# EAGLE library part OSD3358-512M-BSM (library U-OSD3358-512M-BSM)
Octavo Systems LLC OSD335x Family SiP: 21mm x 21mm, 1.27mm pitch 256 pin BGA contains AM3358, 512MB DDR3, TPS65217, TL5209, 4KB EEPROM and passives. Commerical Temperature (case): 0C to 85C.
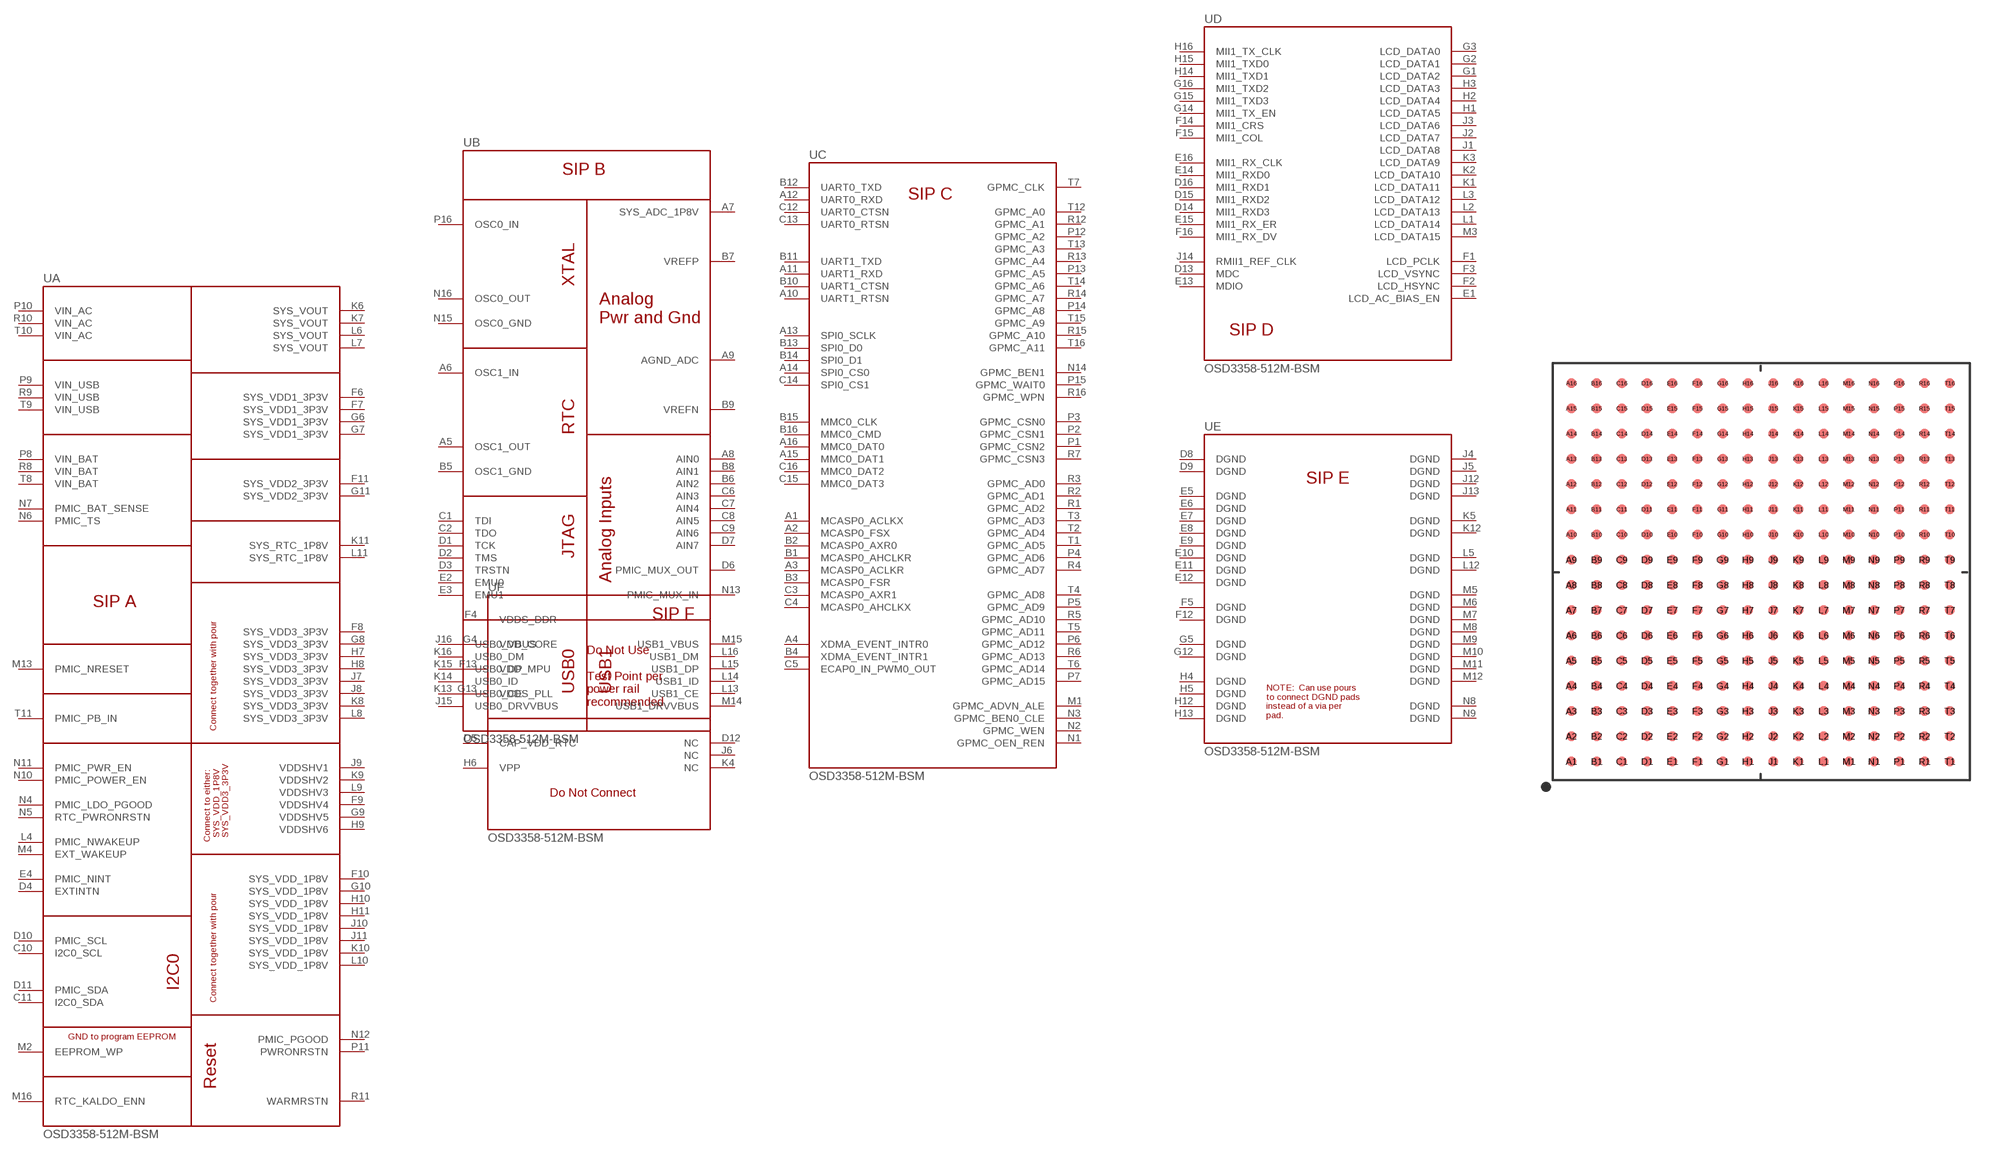
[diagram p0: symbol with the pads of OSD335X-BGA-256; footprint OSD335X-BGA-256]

Designator prefix U; gates A=OSD335X-SM-LOGICAL-A B=OSD335X-SM-LOGICAL-B C=OSD335X-SM-LOGICAL-C D=OSD335X-SM-LOGICAL-D E=OSD335X-SM-LOGICAL-E F=OSD335X-SM-LOGICAL-F

## OSD3358-512M-BSM (DESCRIPTION: 21mm 256 Ball Bga; DIGI-KEY_PART_NUMBER: 1676-1002-ND; DIGI-KEY_PURCHASE_URL: https://www.digikey.com/product-detail/en/octavo-systems-llc/OSD3358-512M-BSM/1676-1002-ND/7644258?utm_source=snapeda&utm_medium=aggregator&utm_campaign=symbol; MF: Octavo Systems; MP: OSD3358-512M-BSM; PACKAGE: BGA-400 Octavo Systems)  [OSD335X-BGA-256]
A1  C:MCASP0_ACLKX
A2  C:MCASP0_FSX
A3  C:MCASP0_ACLKR
A4  C:XDMA_EVENT_INTR0
A5  B:OSC1_OUT
A6  B:OSC1_IN
A7  B:SYS_ADC_1P8V
A8  B:AIN0
A9  B:AGND_ADC
A10  C:UART1_RTSN
A11  C:UART1_RXD
A12  C:UART0_RXD
A13  C:SPI0_SCLK
A14  C:SPI0_CS0
A15  C:MMC0_DAT1
A16  C:MMC0_DAT0
B1  C:MCASP0_AHCLKR
B2  C:MCASP0_AXR0
B3  C:MCASP0_FSR
B4  C:XDMA_EVENT_INTR1
B5  B:OSC1_GND
B6  B:AIN2
B7  B:VREFP
B8  B:AIN1
B9  B:VREFN
B10  C:UART1_CTSN
B11  C:UART1_TXD
B12  C:UART0_TXD
B13  C:SPI0_D0
B14  C:SPI0_D1
B15  C:MMC0_CLK
B16  C:MMC0_CMD
C1  B:TDI
C2  B:TDO
C3  C:MCASP0_AXR1
C4  C:MCASP0_AHCLKX
C5  C:ECAP0_IN_PWM0_OUT
C6  B:AIN3
C7  B:AIN4
C8  B:AIN5
C9  B:AIN6
C10  A:I2C0_SCL
C11  A:I2C0_SDA
C12  C:UART0_CTSN
C13  C:UART0_RTSN
C14  C:SPI0_CS1
C15  C:MMC0_DAT3
C16  C:MMC0_DAT2
D1  B:TCK
D2  B:TMS
D3  B:TRSTN
D4  A:EXTINTN
D5  F:CAP_VDD_RTC
D6  B:PMIC_MUX_OUT
D7  B:AIN7
D8  E:DGND
D9  E:DGND
D10  A:PMIC_SCL
D11  A:PMIC_SDA
D12  F:NC
D13  D:MDC
D14  D:MII1_RXD3
D15  D:MII1_RXD2
D16  D:MII1_RXD1
E1  D:LCD_AC_BIAS_EN
E2  B:EMU0
E3  B:EMU1
E4  A:PMIC_NINT  out
E5  E:DGND
E6  E:DGND
E7  E:DGND
E8  E:DGND
E9  E:DGND
E10  E:DGND
E11  E:DGND
E12  E:DGND
E13  D:MDIO
E14  D:MII1_RXD0
E15  D:MII1_RX_ER
E16  D:MII1_RX_CLK
F1  D:LCD_PCLK
F2  D:LCD_HSYNC
F3  D:LCD_VSYNC
F4  F:VDDS_DDR
F5  E:DGND
F6  A:SYS_VDD1_3P3V  pwr
F7  A:SYS_VDD1_3P3V  pwr
F8  A:SYS_VDD3_3P3V  pwr
F9  A:VDDSHV4  pwr
F10  A:SYS_VDD_1P8V  pwr
F11  A:SYS_VDD2_3P3V  pwr
F12  E:DGND
F13  F:VDD_MPU
F14  D:MII1_CRS
F15  D:MII1_COL
F16  D:MII1_RX_DV
G1  D:LCD_DATA2
G2  D:LCD_DATA1
G3  D:LCD_DATA0
G4  F:VDD_CORE
G5  E:DGND
G6  A:SYS_VDD1_3P3V  pwr
G7  A:SYS_VDD1_3P3V  pwr
G8  A:SYS_VDD3_3P3V  pwr
G9  A:VDDSHV5  pwr
G10  A:SYS_VDD_1P8V  pwr
G11  A:SYS_VDD2_3P3V  pwr
G12  E:DGND
G13  F:VDDS_PLL
G14  D:MII1_TX_EN
G15  D:MII1_TXD3
G16  D:MII1_TXD2
H1  D:LCD_DATA5
H2  D:LCD_DATA4
H3  D:LCD_DATA3
H4  E:DGND
H5  E:DGND
H6  F:VPP
H7  A:SYS_VDD3_3P3V  pwr
H8  A:SYS_VDD3_3P3V  pwr
H9  A:VDDSHV6  pwr
H10  A:SYS_VDD_1P8V  pwr
H11  A:SYS_VDD_1P8V  pwr
H12  E:DGND
H13  E:DGND
H14  D:MII1_TXD1
H15  D:MII1_TXD0
H16  D:MII1_TX_CLK
J1  D:LCD_DATA8
J2  D:LCD_DATA7
J3  D:LCD_DATA6
J4  E:DGND
J5  E:DGND
J6  F:NC
J7  A:SYS_VDD3_3P3V  pwr
J8  A:SYS_VDD3_3P3V  pwr
J9  A:VDDSHV1  pwr
J10  A:SYS_VDD_1P8V  pwr
J11  A:SYS_VDD_1P8V  pwr
J12  E:DGND
J13  E:DGND
J14  D:RMII1_REF_CLK
J15  B:USB0_DRVVBUS
J16  B:USB0_VBUS
K1  D:LCD_DATA11
K2  D:LCD_DATA10
K3  D:LCD_DATA9
K4  F:NC
K5  E:DGND
K6  A:SYS_VOUT  pwr
K7  A:SYS_VOUT  pwr
K8  A:SYS_VDD3_3P3V  pwr
K9  A:VDDSHV2  pwr
K10  A:SYS_VDD_1P8V  pwr
K11  A:SYS_RTC_1P8V  pwr
K12  E:DGND
K13  B:USB0_CE
K14  B:USB0_ID
K15  B:USB0_DP
K16  B:USB0_DM
L1  D:LCD_DATA14
L2  D:LCD_DATA13
L3  D:LCD_DATA12
L4  A:PMIC_NWAKEUP  out
L5  E:DGND
L6  A:SYS_VOUT  pwr
L7  A:SYS_VOUT  pwr
L8  A:SYS_VDD3_3P3V  pwr
L9  A:VDDSHV3  pwr
L10  A:SYS_VDD_1P8V  pwr
L11  A:SYS_RTC_1P8V  pwr
L12  E:DGND
L13  B:USB1_CE
L14  B:USB1_ID
L15  B:USB1_DP
L16  B:USB1_DM
M1  C:GPMC_ADVN_ALE
M2  A:EEPROM_WP
M3  D:LCD_DATA15
M4  A:EXT_WAKEUP
M5  E:DGND
M6  E:DGND
M7  E:DGND
M8  E:DGND
M9  E:DGND
M10  E:DGND
M11  E:DGND
M12  E:DGND
M13  A:PMIC_NRESET
M14  B:USB1_DRVVBUS
M15  B:USB1_VBUS
M16  A:RTC_KALDO_ENN
N1  C:GPMC_OEN_REN
N2  C:GPMC_WEN
N3  C:GPMC_BEN0_CLE
N4  A:PMIC_LDO_PGOOD  out
N5  A:RTC_PWRONRSTN
N6  A:PMIC_TS
N7  A:PMIC_BAT_SENSE
N8  E:DGND
N9  E:DGND
N10  A:PMIC_POWER_EN  out
N11  A:PMIC_PWR_EN  in
N12  A:PMIC_PGOOD  out
N13  B:PMIC_MUX_IN
N14  C:GPMC_BEN1
N15  B:OSC0_GND
N16  B:OSC0_OUT
P1  C:GPMC_CSN2
P2  C:GPMC_CSN1
P3  C:GPMC_CSN0
P4  C:GPMC_AD6
P5  C:GPMC_AD9
P6  C:GPMC_AD12
P7  C:GPMC_AD15
P8  A:VIN_BAT  pwr
P9  A:VIN_USB  pwr
P10  A:VIN_AC  pwr
P11  A:PWRONRSTN
P12  C:GPMC_A2
P13  C:GPMC_A5
P14  C:GPMC_A8
P15  C:GPMC_WAIT0
P16  B:OSC0_IN
R1  C:GPMC_AD2
R2  C:GPMC_AD1
R3  C:GPMC_AD0
R4  C:GPMC_AD7
R5  C:GPMC_AD10
R6  C:GPMC_AD13
R7  C:GPMC_CSN3
R8  A:VIN_BAT  pwr
R9  A:VIN_USB  pwr
R10  A:VIN_AC  pwr
R11  A:WARMRSTN
R12  C:GPMC_A1
R13  C:GPMC_A4
R14  C:GPMC_A7
R15  C:GPMC_A10
R16  C:GPMC_WPN
T1  C:GPMC_AD5
T2  C:GPMC_AD4
T3  C:GPMC_AD3
T4  C:GPMC_AD8
T5  C:GPMC_AD11
T6  C:GPMC_AD14
T7  C:GPMC_CLK
T8  A:VIN_BAT  pwr
T9  A:VIN_USB  pwr
T10  A:VIN_AC  pwr
T11  A:PMIC_PB_IN
T12  C:GPMC_A0
T13  C:GPMC_A3
T14  C:GPMC_A6
T15  C:GPMC_A9
T16  C:GPMC_A11

## Footprint OSD335X-BGA-256 (pad centres in mm)
smd 0.5 x 0.5: A1 -9.525,-9.525; A2 -9.525,-8.255; A3 -9.525,-6.985; A4 -9.525,-5.715; A5 -9.525,-4.445; A6 -9.525,-3.175; A7 -9.525,-1.905; A8 -9.525,-0.635; A9 -9.525,0.635; A10 -9.525,1.905; A11 -9.525,3.175; A12 -9.525,4.445; A13 -9.525,5.715; A14 -9.525,6.985; A15 -9.525,8.255; A16 -9.525,9.525; B1 -8.255,-9.525; B2 -8.255,-8.255; B3 -8.255,-6.985; B4 -8.255,-5.715; B5 -8.255,-4.445; B6 -8.255,-3.175; B7 -8.255,-1.905; B8 -8.255,-0.635; B9 -8.255,0.635; B10 -8.255,1.905; B11 -8.255,3.175; B12 -8.255,4.445; B13 -8.255,5.715; B14 -8.255,6.985; B15 -8.255,8.255; B16 -8.255,9.525; C1 -6.985,-9.525; C2 -6.985,-8.255; C3 -6.985,-6.985; C4 -6.985,-5.715; C5 -6.985,-4.445; C6 -6.985,-3.175; C7 -6.985,-1.905; C8 -6.985,-0.635; C9 -6.985,0.635; C10 -6.985,1.905; C11 -6.985,3.175; C12 -6.985,4.445; C13 -6.985,5.715; C14 -6.985,6.985; C15 -6.985,8.255; C16 -6.985,9.525; D1 -5.715,-9.525; D2 -5.715,-8.255; D3 -5.715,-6.985; D4 -5.715,-5.715; D5 -5.715,-4.445; D6 -5.715,-3.175; D7 -5.715,-1.905; D8 -5.715,-0.635; D9 -5.715,0.635; D10 -5.715,1.905; D11 -5.715,3.175; D12 -5.715,4.445; D13 -5.715,5.715; D14 -5.715,6.985; D15 -5.715,8.255; D16 -5.715,9.525; E1 -4.445,-9.525; E2 -4.445,-8.255; E3 -4.445,-6.985; E4 -4.445,-5.715; E5 -4.445,-4.445; E6 -4.445,-3.175; E7 -4.445,-1.905; E8 -4.445,-0.635; E9 -4.445,0.635; E10 -4.445,1.905; E11 -4.445,3.175; E12 -4.445,4.445; E13 -4.445,5.715; E14 -4.445,6.985; E15 -4.445,8.255; E16 -4.445,9.525; F1 -3.175,-9.525; F2 -3.175,-8.255; F3 -3.175,-6.985; F4 -3.175,-5.715; F5 -3.175,-4.445; F6 -3.175,-3.175; F7 -3.175,-1.905; F8 -3.175,-0.635; F9 -3.175,0.635; F10 -3.175,1.905; F11 -3.175,3.175; F12 -3.175,4.445; F13 -3.175,5.715; F14 -3.175,6.985; F15 -3.175,8.255; F16 -3.175,9.525; G1 -1.905,-9.525; G2 -1.905,-8.255; G3 -1.905,-6.985; G4 -1.905,-5.715; G5 -1.905,-4.445; G6 -1.905,-3.175; G7 -1.905,-1.905; G8 -1.905,-0.635; G9 -1.905,0.635; G10 -1.905,1.905; G11 -1.905,3.175; G12 -1.905,4.445; G13 -1.905,5.715; G14 -1.905,6.985; G15 -1.905,8.255; G16 -1.905,9.525; H1 -0.635,-9.525; H2 -0.635,-8.255; H3 -0.635,-6.985; H4 -0.635,-5.715; H5 -0.635,-4.445; H6 -0.635,-3.175; H7 -0.635,-1.905; H8 -0.635,-0.635; H9 -0.635,0.635; H10 -0.635,1.905; H11 -0.635,3.175; H12 -0.635,4.445; H13 -0.635,5.715; H14 -0.635,6.985; H15 -0.635,8.255; H16 -0.635,9.525; J1 0.635,-9.525; J2 0.635,-8.255; J3 0.635,-6.985; J4 0.635,-5.715; J5 0.635,-4.445; J6 0.635,-3.175; J7 0.635,-1.905; J8 0.635,-0.635; J9 0.635,0.635; J10 0.635,1.905; J11 0.635,3.175; J12 0.635,4.445; J13 0.635,5.715; J14 0.635,6.985; J15 0.635,8.255; J16 0.635,9.525; K1 1.905,-9.525; K2 1.905,-8.255; K3 1.905,-6.985; K4 1.905,-5.715; K5 1.905,-4.445; K6 1.905,-3.175; K7 1.905,-1.905; K8 1.905,-0.635; K9 1.905,0.635; K10 1.905,1.905; K11 1.905,3.175; K12 1.905,4.445; K13 1.905,5.715; K14 1.905,6.985; K15 1.905,8.255; K16 1.905,9.525; L1 3.175,-9.525; L2 3.175,-8.255; L3 3.175,-6.985; L4 3.175,-5.715; L5 3.175,-4.445; L6 3.175,-3.175; L7 3.175,-1.905; L8 3.175,-0.635; L9 3.175,0.635; L10 3.175,1.905; L11 3.175,3.175; L12 3.175,4.445; L13 3.175,5.715; L14 3.175,6.985; L15 3.175,8.255; L16 3.175,9.525; M1 4.445,-9.525; M2 4.445,-8.255; M3 4.445,-6.985; M4 4.445,-5.715; M5 4.445,-4.445; M6 4.445,-3.175; M7 4.445,-1.905; M8 4.445,-0.635; M9 4.445,0.635; M10 4.445,1.905; M11 4.445,3.175; M12 4.445,4.445; M13 4.445,5.715; M14 4.445,6.985; M15 4.445,8.255; M16 4.445,9.525; N1 5.715,-9.525; N2 5.715,-8.255; N3 5.715,-6.985; N4 5.715,-5.715; N5 5.715,-4.445; N6 5.715,-3.175; N7 5.715,-1.905; N8 5.715,-0.635; N9 5.715,0.635; N10 5.715,1.905; N11 5.715,3.175; N12 5.715,4.445; N13 5.715,5.715; N14 5.715,6.985; N15 5.715,8.255; N16 5.715,9.525; P1 6.985,-9.525; P2 6.985,-8.255; P3 6.985,-6.985; P4 6.985,-5.715; P5 6.985,-4.445; P6 6.985,-3.175; P7 6.985,-1.905; P8 6.985,-0.635; P9 6.985,0.635; P10 6.985,1.905; P11 6.985,3.175; P12 6.985,4.445; P13 6.985,5.715; P14 6.985,6.985; P15 6.985,8.255; P16 6.985,9.525; R1 8.255,-9.525; R2 8.255,-8.255; R3 8.255,-6.985; R4 8.255,-5.715; R5 8.255,-4.445; R6 8.255,-3.175; R7 8.255,-1.905; R8 8.255,-0.635; R9 8.255,0.635; R10 8.255,1.905; R11 8.255,3.175; R12 8.255,4.445; R13 8.255,5.715; R14 8.255,6.985; R15 8.255,8.255; R16 8.255,9.525; T1 9.525,-9.525; T2 9.525,-8.255; T3 9.525,-6.985; T4 9.525,-5.715; T5 9.525,-4.445; T6 9.525,-3.175; T7 9.525,-1.905; T8 9.525,-0.635; T9 9.525,0.635; T10 9.525,1.905; T11 9.525,3.175; T12 9.525,4.445; T13 9.525,5.715; T14 9.525,6.985; T15 9.525,8.255; T16 9.525,9.525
